FUNCTION_BLOCK FileExample02_ReadLogs //any combination of flyways and xbots - GetErrorLog, GetWarningLog. Any existing 'warning_log.txt' or 'error_log.txt' file in DemoFilesFolder will be overwritten
VAR_INPUT
	Execute : BOOL;
	DemoFilesFolder : STRING(255);	//Folder that contains the GCodeDemo.txt file
END_VAR
VAR_OUTPUT
	Done : BOOL;
END_VAR
VAR_IN_OUT
	PM_Controller : PMControllerType;	// the planar motor controller to use
END_VAR
VAR
	PMC_GetWarningLog1 : PMC_GetWarningLog;	
	warninglog : ARRAY[0..99999] OF SINT;
	write_warning_log : WriteFileOnDisk;
	PMC_GetErrorLog1 : PMC_GetErrorLog;
	errorlog : ARRAY[0..99999] OF SINT;
	write_error_log : WriteFileOnDisk;	
END_VAR

//any combination of flyways and xbots - GetErrorLog, GetWarningLog
//Any existing 'warning_log.txt' or 'error_log.txt' file in DemoFilesFolder will be overwritten

//get the PMC warning log
PMC_GetWarningLog1(Execute := Execute,Bytes := warninglog,PM_Controller := PM_Controller);

//write the warning log to disk
write_warning_log(Execute := PMC_GetWarningLog1.Done,file_path := CONCAT(STR1 := DemoFilesFolder,STR2 := '\warning_log.txt'),file_size := PMC_GetWarningLog1.nBytes,data := warninglog);

//get the PMC error log
PMC_GetErrorLog1(Execute := write_warning_log.Done,Bytes := errorlog,PM_Controller := PM_Controller);

//write the error log to disk
write_error_log(Execute := PMC_GetErrorLog1.Done,file_path := CONCAT(STR1 := DemoFilesFolder,STR2 := '\error_log.txt'),file_size := PMC_GetErrorLog1.nBytes,data := errorlog);

Done := write_error_log.Done;

END_FUNCTION_BLOCK
